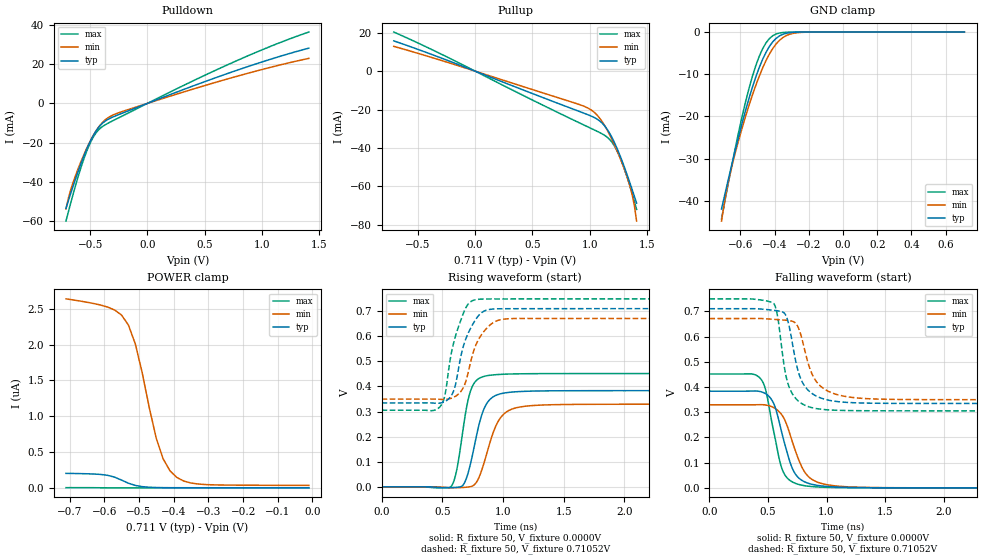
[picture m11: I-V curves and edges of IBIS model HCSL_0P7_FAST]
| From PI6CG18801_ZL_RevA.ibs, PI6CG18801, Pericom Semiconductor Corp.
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[Model]   HCSL_0P7_FAST
Model_type Output
Vref=0.7000V
Vmeas=900mV
| variable   typ   min   max
C_comp   2.000pF   1.970pF   2.030pF
[Voltage Range]   0.71052V   0.67147V   0.74949V
[POWER Clamp Reference]   0.71052V   0.67147V   0.74949V
[GND Clamp Reference]   0.0000V   0.0000V   0.0000V
[Pullup Reference]   0.71052V   0.67147V   0.74949V
[Pulldown Reference]   0.0000V   0.0000V   0.0000V
[Temperature Range]   25   85   -40
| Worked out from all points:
|   slope of the pulldown table from 0 to 0.107 V, typ, clamps not added: 43.9 ohm
|   slope of the pullup table from 0 to 0.107 V, typ, clamps not added: 42.4 ohm
|   GND clamp passes 1 mA (typ) near -0.37 V on its own axis
|   falling waveform, R_fixture 50, V_fixture 0.0000V: 20-80 % time 138ps typ, 160ps min, 116ps max; typ from 0.384 V to 0 V
|   rising waveform, R_fixture 50, V_fixture 0.0000V: 20-80 % time 115ps typ, 139ps min, 92ps max; typ from 0 V to 0.383 V
|   falling waveform, R_fixture 50, V_fixture 0.71052V: 20-80 % time 121ps typ, 146ps min, 97ps max; typ from 0.711 V to 0.335 V
|   rising waveform, R_fixture 50, V_fixture 0.71052V: 20-80 % time 126ps typ, 134ps min, 118ps max; typ from 0.335 V to 0.711 V
[GND Clamp]
| Voltage   I(typ)   I(min)   I(max)
-710.5mV  -41.93mA   -44.79mA   -44.29mA
-690.5mV  -38.38mA   -39.63mA   -39.99mA
-650.5mV  -31.43mA   -31.94mA   -31.6mA
-590.5mV  -21.65mA   -22.79mA   -20.07mA
-550.5mV  -15.81mA   -17.46mA   -13.46mA
-510.5mV  -10.7mA    -12.68mA   -8.013mA
-470.5mV  -6.503mA   -8.547mA   -3.986mA
-450.5mV  -4.807mA   -6.77mA    -2.569mA
-410.5mV  -2.292mA   -3.877mA   -863uA
-350.5mV  -515.2uA   -1.274mA   -104.6uA
-250.5mV  -20.58uA   -103.2uA   -1.252uA
709.5mV   1.155nA    34.32nA    -1.818pA
[POWER Clamp]
| Voltage   I(typ)   I(min)   I(max)
-710.5mV  202.2nA    2.638uA    2.798nA
-570.5mV  149.4nA    2.483uA    234pA
-550.5mV  108.7nA    2.413uA    105.5pA
-530.5mV  64.8nA     2.273uA    56.58pA
-510.5mV  33.41nA    2.008uA    37.69pA
-490.5mV  16.56nA    1.601uA    30.01pA
-450.5mV  4.682nA    697nA      24.52pA
-430.5mV  2.929nA    406.3nA    23.13pA
-410.5mV  2.112nA    236.4nA    21.95pA
-390.5mV  1.728nA    143.6nA    20.85pA
-310.5mV  1.373nA    46.52nA    16.62pA
-10.52mV  1.163nA    33.88nA    840fA
[Pulldown]
| Voltage   I(typ)   I(min)   I(max)
-710.5mV  -53.57mA   -53.89mA   -60.08mA
-690.5mV  -49.91mA   -48.65mA   -55.62mA
-650.5mV  -42.7mA    -40.76mA   -46.88mA
-550.5mV  -26.33mA   -25.71mA   -27.7mA
-510.5mV  -20.85mA   -20.65mA   -21.72mA
-470.5mV  -16.23mA   -16.21mA   -17.05mA
-410.5mV  -11.21mA   -10.96mA   -12.68mA
-350.5mV  -8.379mA   -7.605mA   -10.34mA
-290.5mV  -6.678mA   -5.686mA   -8.527mA
69.48mV   1.588mA    1.304mA    2.051mA
809.5mV   17.48mA    14.31mA    22.58mA
1.409V    28.24mA    23mA       36.47mA
[Pullup]
| Voltage   I(typ)   I(min)   I(max)
-710.5mV  15.78mA    12.92mA    20.39mA
869.5mV   -20.11mA   -16.62mA   -25.8mA
1.029V    -23.88mA   -20.96mA   -30.35mA
1.069V    -25.19mA   -23.25mA   -31.49mA
1.129V    -28.46mA   -28.28mA   -33.44mA
1.189V    -34.06mA   -35.02mA   -36.69mA
1.229V    -39.02mA   -40.24mA   -40.46mA
1.289V    -47.89mA   -49.02mA   -48.79mA
1.349V    -57.98mA   -59.53mA   -59.62mA
1.369V    -61.53mA   -64.06mA   -63.63mA
1.389V    -65.14mA   -69.88mA   -67.8mA
1.409V    -68.79mA   -78.13mA   -72.1mA
[Falling Waveform]
R_fixture = 50
V_fixture = 0.0000V
V_fixture_min = 0.0000V
V_fixture_max = 0.0000V
|   Time   V(typ)   V(min)   V(max)
0s        383.5mV    329.4mV    451.7mV
440ps     381.2mV    329.9mV    431.2mV
480ps     373.4mV    328.6mV    389.2mV
540ps     342.9mV    320.3mV    243.7mV
620ps     215.1mV    288.4mV    74.96mV
710ps     74.92mV    180.3mV    22.92mV
790ps     29.58mV    82.03mV    10.44mV
920ps     9.979mV    22.98mV    3.612mV
1.2ns     1.611mV    3.748mV    567.9uV
5ns       19.75uV    21.03uV    18.57uV
[Rising Waveform]
R_fixture = 50
V_fixture = 0.0000V
V_fixture_min = 0.0000V
V_fixture_max = 0.0000V
|   Time   V(typ)   V(min)   V(max)
0s        9.257uV    9.884uV    9.331uV
570ps     -3.337mV   -3.911mV   -160.3uV
620ps     -2.042mV   -3.705mV   70.41mV
680ps     13.67mV    -2.307mV   258.9mV
730ps     87.53mV    443.8uV    378.9mV
790ps     222.6mV    25.37mV    428.2mV
870ps     335.2mV    139.3mV    443.2mV
990ps     372.1mV    281.8mV    448.6mV
1.2ns     381.1mV    322.3mV    450.9mV
5ns       383.5mV    329.4mV    451.7mV
[Falling Waveform]
R_fixture = 50
V_fixture = 0.71052V
V_fixture_min = 0.67147V
V_fixture_max = 0.74949V
|   Time   V(typ)   V(min)   V(max)
0s        710.5mV    671.5mV    749.5mV
550ps     704.1mV    668.4mV    730.8mV
580ps     702.5mV    667.3mV    685.5mV
640ps     693mV      665.3mV    478.4mV
680ps     643.2mV    663.4mV    400.5mV
770ps     444.4mV    622.6mV    340.2mV
910ps     364.7mV    423.6mV    314.7mV
1.08ns    342.9mV    371.2mV    307.8mV
1.38ns    335.8mV    353mV      305.8mV
5ns       334.7mV    349.7mV    305.4mV
[Rising Waveform]
R_fixture = 50
V_fixture = 0.71052V
V_fixture_min = 0.67147V
V_fixture_max = 0.74949V
|   Time   V(typ)   V(min)   V(max)
0s        334.6mV    349.7mV    305.4mV
480ps     333.8mV    348.8mV    318.9mV
520ps     339.6mV    348.4mV    361.5mV
580ps     368.5mV    354.1mV    546.7mV
630ps     461.1mV    368.6mV    633.8mV
690ps     585.2mV    414.9mV    710.5mV
780ps     671.1mV    569.7mV    746.6mV
900ps     708mV      648.1mV    749mV
1.04ns    710.2mV    670.1mV    749.2mV
5ns       710.5mV    671.4mV    749.5mV
[Ramp]
| variable   typ   min   max
dV/dt_r   0.22989V/115.34p   0.19737V/139.06p   0.27088V/91.995p
dV/dt_f   0.22534V/121.45p   0.19298V/146.10p   0.26597V/96.990p
R_load = 50
